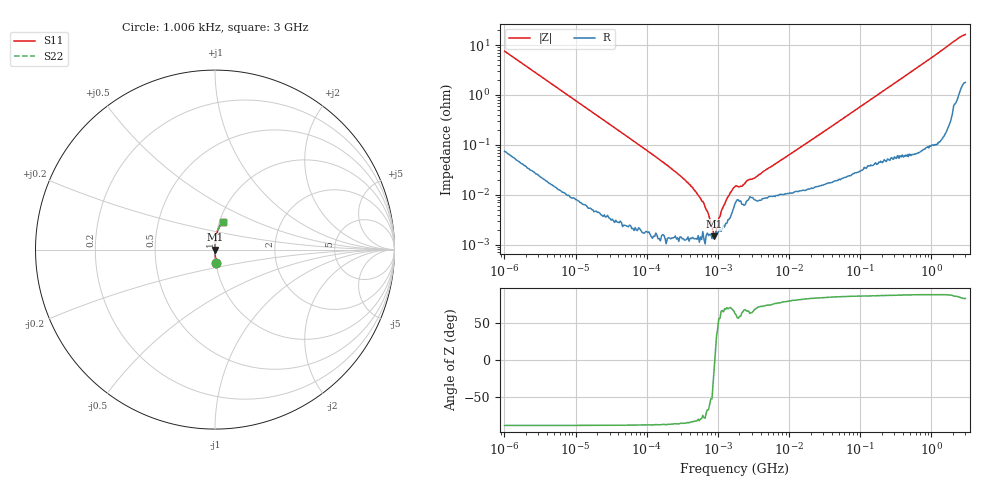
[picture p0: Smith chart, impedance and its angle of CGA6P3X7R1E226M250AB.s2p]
! S-Parameter Data Generated by TDK Corporation
! Copyright(C) 2020 TDK Corporation.
! All Rights Reserved.
! TDK P/N: CGA6P3X7R1E226M250AB (Multilayer Ceramic Chip Capacitor)
! Property: C=22uF
! Size(LxWxT): 3.2x2.5x2.5mm
! Model Type: s2p (Touchstone File Format Version 1.0)
! Frequency: DC=Yes Start=0.001006039MHz Stop=3000MHz 480points Log-sweep
! Model Generated on Nov. 18, 2020
! Port Assignments:
!  1 ---| |--- 2
! Applicable Conditions:
!  Temperature = 25 degC
!  DC Bias Voltage = 0 V
!  Small Signal Operation
! Terms and conditions regarding TDK Simulation Models
! (1)This simulation model is being provided solely for informational purposes. Please refer to the specifications of the products in terms of detailed characteristics of such products.
! (2)In no event shall TDK Corporation of any of its subsidiaries be liable for any loss or damage arising, directly or indirectly,
!  From any information contained in this simulation model, including, but not limited to loss or damages arising from any inaccuracies, omissions or errors in connection with such information.
! (3)Any and all copyrights on this simulation model are owned by TDK Corporation.
!  Duplication or redistribution of this simulation model without prior written permission from TDK Corporation is prohibited.
! (4)This simulation model is subject to any modification or change without any prior notice.
! (5)Neither TDK Corporation nor any of its subsidiaries shall make any warranty, express or implied,
!  Including but not limited to the correctness, implied warranties of merchantability and fitness for a particular purpose with respect to this simulation models.
! (6)The use of this simulation model shall be deemed to have consented to the terms and conditions hereof.
# Hz S MA R 50
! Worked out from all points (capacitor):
!   479 points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, 1.006 kHz to 3 GHz, reference 50 ohm
!   read as one part in series: C = 20.9 uF near 1.083 kHz
!   lowest |Z| = 1.46 mohm at 888.4 kHz (marker M1)
!   series resonance near 905.3 kHz, so ESL is about 1.5 nH
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1006.039  0.07511 -85.1  0.9964 4.3  0.9964 4.3  0.07511 -85.1
2840.326  0.02694 -87.9  0.9994 1.5  0.9994 1.5  0.02694 -87.9
12511.27  0.006179 -89.1  0.9999 0.4  0.9999 0.4  0.006179 -89.1
149930.4  0.000509 -88.5  1 0.0  1 0.0  0.000509 -88.5
314670.7  0.0002194 -86.6  1 0.0  1 0.0  0.0002194 -86.6
407891.4  0.0001562 -85.0  1 0.0  1 0.0  0.0001562 -85.0
528728.7  9.763e-05 -81.1  1 0.0  1 0.0  9.763e-05 -81.1
569415.9  8.432e-05 -80.3  1 0.0  1 0.0  8.432e-05 -80.3
888402.1  1.458e-05 -10.6  1 0.0  1 0.0  1.458e-05 -10.6
1386084  9.068e-05 69.7  1 -0.0  1 -0.0  9.068e-05 69.7
1492747  0.0001101 71.5  1 -0.0  1 -0.0  0.0001101 71.5
1668327  0.0001387 66.8  0.9999 -0.0  0.9999 -0.0  0.0001387 66.8
1796709  0.0001519 61.5  0.9999 -0.0  0.9999 -0.0  0.0001519 61.5
2083873  0.0001483 59.5  0.9999 -0.0  0.9999 -0.0  0.0001483 59.5
2701217  0.0001982 66.5  0.9999 -0.0  0.9999 -0.0  0.0001982 66.5
3374034  0.0002227 69.6  0.9999 -0.0  0.9999 -0.0  0.0002227 69.6
4538749  0.0003043 73.9  0.9999 -0.0  0.9999 -0.0  0.0003043 73.9
2.153109e7  0.001306 84.1  0.9999 -0.1  0.9999 -0.1  0.001306 84.1
2.507343e8  0.01423 87.2  0.9994 -0.8  0.9994 -0.8  0.01423 87.2
1.017911e9  0.05652 85.8  0.9974 -3.2  0.9974 -3.2  0.05652 85.8
2.359433e9  0.1332 78.6  0.9823 -7.6  0.9823 -7.6  0.1332 78.6
3e9  0.1584 74.7  0.9703 -9.1  0.9703 -9.1  0.1584 74.7
